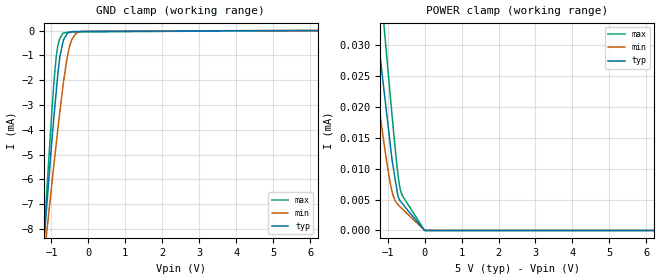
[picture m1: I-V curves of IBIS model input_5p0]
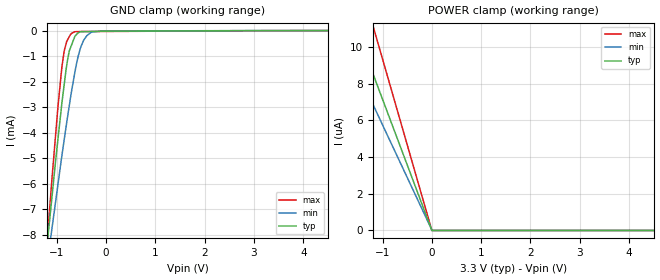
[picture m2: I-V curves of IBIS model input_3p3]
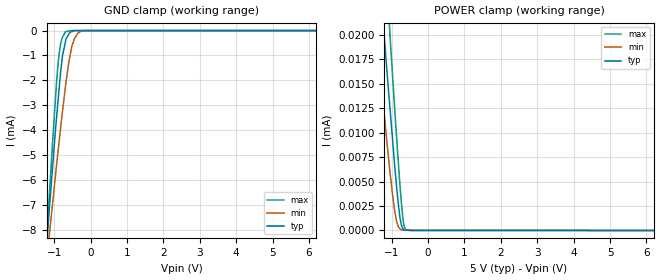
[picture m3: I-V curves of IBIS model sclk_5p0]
|Texas Instruments Incorporated
| 3 Phase Motor Driver-IC for Automotive Safety Applications
| Marketing part#   Digital Voltage Range   Package-type   #pins
| DRV3201QPAPQ1   1.72V-5.5V   HTQFP   64
[IBIS Ver]   4.1
[File name]   drv3201.ibs
[File Rev]   1.0
[Date]   2/26/2013
[Source]
| Texas Instruments Incorporated.
| Analog-eLab Design Center, HPA
| 12500 TI Blvd
| Dallas, TX -75243
[Notes]   Revision History:
| Rev 1.0: 2/26/2013
| - Initial version of the model
| - Model generated from simulations in TISPICE
| - Model matched to SPICE simulation
| - C_comp although listed in numerical order of value are
|   obtained from varying PVT conditions. For PVT conditions for
|   each specific value refer the buffer description under
|   respective [Model]. IBIS model user is responsible for using
|   appropriate C_comp to simulate for Signal Integrity.
| - Model names with a trailing _3p3 contains the model for 3.3V
|   [3.0V and 3.6V]. Model names with a trailing _5 contains the
|   model for 5.0V [4.5V and 5.5V].
[Disclaimer]
| This model is designed as an aid for customers of Texas Instruments.
| TI and its licensors and suppliers make no warranties, either expressed
| or implied, with respect to this  model, including the warranties of
| merchantability or fitness for a particular purpose. The model is
| provided solely on an "as is" basis. The entire risk as to its quality
| and performance is with the customer.
|*  EXCEPTION:   *
|*  - For model en_*, there will be a leakage current in the power clamp   *
|*   I-V Table because of the pull down resistor RES_P1H (200K) and the   *
|*   diode DIO_Z_CB_MV1 connected to pad.   *
|*  - For model input_*, there will be a leakage current in the ground   *
|*   clamp I-V Table because of the  pull-up resistor RES_P1H (140K)   *
|*   connected to pad.   *
|*  - For model sclk_*, there will be a leakage current in the power clamp  *
|*   I-V Table because of the esd transistor NPN_ESD_5A connected to pad.  *
|*  - For model sdi_*, there will be a leakage current in the power clamp   *
|*   I-V Table because of the esd transistor NPN_ESD_5A connected to pad.  *
[Copyright]
(C) Copyright 2013 Texas Instruments Incorporated.All rights reserved.
|   DRV3201
[Component]   DRV3201
[Manufacturer]   TI
[Package]   |64 HTQFP   -  PAP package
|   typ   min   max
R_pkg   0.07164   0.06786   0.07759
L_pkg   3.33226nH   3.17288nH   3.57776nH
C_pkg   0.48700pF   0.46154pF   0.50805pF
[Pin]  signal_name   model_name   R_pin   L_pin   C_pin
1   VSH   NC   0.07673   3.54889nH  0.46840pF
2   SLS3   POWER   0.07311   3.39626nH  0.51137pF
3   GLS3   POWER   0.07001   3.27956nH  0.49926pF
4   SHS3   POWER   0.06923   3.24062nH  0.49391pF
5   GHS3   POWER   0.06747   3.17175nH  0.48377pF
6   PGND   GND   0.06709   3.14589nH  0.47600pF
7   SLS2   POWER   0.06644   3.11361nH  0.47461pF
8   GLS2   POWER   0.06615   3.10081nH  0.46390pF
9   SHS2   POWER   0.06619   3.10253nH  0.46433pF
10   GHS2   POWER   0.06676   3.12576nH  0.48040pF
11   GNDA   GND   0.06824   3.18796nH  0.48872pF
12   SCTH   NC   0.07010   3.26538nH  0.49431pF
13   SLS1   POWER   0.07197   3.33861nH  0.50666pF
14   GLS1   POWER   0.07533   3.46841nH  0.51599pF
15   SHS1   POWER   0.07680   3.52858nH  0.52091pF
16   GHS1   POWER   0.08171   3.72851nH  0.48358pF
17   PH1C   PH   0.07690   3.56798nH  0.46154pF
18   PH2C   PH   0.07539   3.49007nH  0.50339pF
19   PH3C   PH   0.07491   3.46547nH  0.50805pF
20   GNDA   GND   0.07195   3.34941nH  0.50551pF
21   DRVOFF   INPUT   0.06967   3.26125nH  0.48761pF
22   SCLK   SCLK   0.06998   3.25832nH  0.48236pF
23   GNDL   GND   0.06864   3.20087nH  0.48096pF
24   NCS   INPUT   0.06798   3.17337nH  0.46659pF
25   SDI   SDI   0.06796   3.17288nH  0.46520pF
26   SDO   SDO   0.06786   3.17339nH  0.47390pF
27   GNDA   GND   0.06804   3.19040nH  0.48153pF
28   VS   POWER   0.06907   3.23961nH  0.48931pF
29   BOOST   POWER   0.06978   3.27269nH  0.49651pF
30   SW   POWER   0.03802   3.09902nH  0.55354pF
31   GNDLS_B   GND   0.03874   3.15006nH  0.56153pF
32   NC   NC   0.07644   3.55028nH  0.47304pF
33   NC   NC   0.07611   3.53711nH  0.46336pF
34   B_EN   INPUT   0.07412   3.44194nH  0.50787pF
35   CSM   SDI   0.07078   3.31667nH  0.49695pF
36   EN   EN   0.07096   3.31071nH  0.49365pF
37   RSTN   INPUT   0.06872   3.22236nH  0.48158pF
38   ERR   ERR   0.07110   3.29339nH  0.48566pF
39   GNDA   GND   0.06849   3.19000nH  0.48290pF
40   VCC5   NC   0.06688   3.12853nH  0.46693pF
41   TEST(GND)   NC   0.06665   3.11990nH  0.46778pF
42   VCC3   NC   0.03537   2.85634nH  0.51702pF
43   AMUX(GND)   GND   0.06623   3.11968nH  0.47403pF
44   ADREF   NC   0.06627   3.13372nH  0.48099pF
45   GNDL   GND   0.06693   3.16429nH  0.48921pF
46   O4   NC   0.06838   3.22606nH  0.49485pF
47   O3   NC   0.07039   3.30331nH  0.50075pF
48   O2   NC   0.07861   3.61686nH  0.47279pF
49   IN2   NC   0.08054   3.68122nH  0.47742pF
50   IP2   NC   0.07690   3.52768nH  0.52252pF
51   GNDA   GND   0.07282   3.37580nH  0.51523pF
52   RO   NC   0.06992   3.26214nH  0.50012pF
53   RI   NC   0.06865   3.20956nH  0.48695pF
54   IP1   NC   0.06779   3.16608nH  0.47853pF
55   O1   NC   0.06756   3.14757nH  0.47304pF
56   IN1   NC   0.06757   3.14359nH  0.46926pF
57   GNDA   GND   0.06819   3.16549nH  0.47185pF
58   VDDIO   POWER   0.06871   3.18793nH  0.47574pF
59   IHS3   SDI   0.06892   3.20623nH  0.47992pF
60   ILS3   SDI   0.07066   3.28064nH  0.48755pF
61   IHS2   SDI   0.07071   3.29082nH  0.49336pF
62   ILS2   SDI   0.07325   3.39194nH  0.50262pF
63   IHS1   SDI   0.07376   3.41784nH  0.50532pF
64   ILS1   SDI   0.07759   3.57776nH  0.46991pF
|   Model Selectors
[Model Selector] INPUT
input_3p3  3.3V digital input
input_5p0  5.0V digital input
[Model Selector] SCLK
sclk_3p3  3.3V digital input
sclk_5p0  5.0V digital input
[Model Selector] SDI
sdi_3p3  3.3V digital input
sdi_5p0  5.0V digital input
[Model Selector] EN
en_3p3  3.3V digital input
en_5p0  5.0V digital input
[Model Selector] PH
ph_3p3  3.3V digital output
ph_5p0  5.0V digital output
[Model Selector] ERR
err_3p3  3.3V digital output
err_5p0  5.0V digital output
[Model Selector] SDO
sdo_3p3  3.3V digital output
sdo_5p0  5.0V digital output
| Models and submodels in the file (14): input_5p0 (Input), input_3p3 (Input), sclk_5p0 (Input), sclk_3p3 (Input), en_5p0 (Input), en_3p3 (Input), sdi_5p0 (Input), sdi_3p3 (Input), ph_5p0 (Output), ph_3p3 (Output), err_5p0 (Output), err_3p3 (Output), sdo_5p0 (Output), sdo_3p3 (Output)
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|   input_5p0 Model
[Model]   input_5p0
Model_type   Input
Vinl = 1.5
Vinh = 3.5
|   typ   min   max
|   (nom PVT)   (fast PVT)   (slow PVT)
C_comp   4.496e-13   4.401e-13   4.837e-13
| Where nom  PVT is Nominal Process, 5V, 27C
|   Fast PVT is Strong Process,  5.5V, -40C
|   Slow PVT is Weak Process,   4.5V, 150C
[Voltage Range]   5   4.5   5.5
[Temperature Range]   27   150   -40
[Power Clamp Reference]   5   4.5   5.5
[GND Clamp Reference]   0   0   0
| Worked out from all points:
|   GND clamp passes 1 mA (typ) near -0.76 V on its own axis
[GND Clamp]
|   Voltage   I(typ)   I(min)   I(max)
-5V       -87.91mA   -68.74mA   -109.8mA
-1.21V    -8.701mA   -9.359mA   -8.617mA
-1.139V   -7.31mA    -8.314mA   -6.835mA
-1.083V   -6.272mA   -7.533mA   -5.494mA
-940.5mV  -3.622mA   -5.516mA   -2.263mA
-869mV    -2.453mA   -4.558mA   -1.045mA
-770mV    -1.039mA   -3.255mA   -318.7uA
-687.5mV  -468.2uA   -2.242mA   -104.3uA
-513mV    -80.01uA   -652.5uA   -56.2uA
-346.5mV  -38.89uA   -131.6uA   -54.55uA
-202.5mV  -37.57uA   -32.73uA   -53.21uA
10V       0A         0A         0A
[POWER Clamp]
|   Voltage   I(typ)   I(min)   I(max)
-5V       244.6uA    202.3uA    308.1uA
-1.566V   48.38uA    35.32uA    65.5uA
-1.373V   37.57uA    26.3uA     51.98uA
-1.175V   26.68uA    17.38uA    38.37uA
-1.098V   22.63uA    14.09uA    33.11uA
-1.078V   21.59uA    13.27uA    31.73uA
-891mV    11.91uA    6.548uA    19.26uA
-720mV    5.513uA    4.176uA    9.035uA
-671mV    4.865uA    3.873uA    6.977uA
-594mV    4.287uA    3.425uA    5.569uA
-84.44fV  0A         25.24nA    0A
10V       0A         0A         0A
|   input_3p3 Model
[Model]   input_3p3
Model_type   Input
Vinl = 0.99
Vinh = 2.31
|   typ   min   max
|   (nom PVT)   (fast PVT)   (slow PVT)
C_comp   4.837e-13   4.556e-13   5.145e-13
| Where nom  PVT is Nominal Process, 3.3V, 27C
|   Fast PVT is Strong Process,  3.6V, -40C
|   Slow PVT is Weak Process,   3V, 150C
[Voltage Range]   3.3   3   3.6
|Junction Temperature
[Temperature Range]   27   150   -40
[Power Clamp Reference]   3.3   3   3.6
[GND Clamp Reference]   0   0   0
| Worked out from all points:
|   GND clamp passes 1 mA (typ) near -0.77 V on its own axis
[GND Clamp]
|   Voltage   I(typ)   I(min)   I(max)
-3.3V     -51.91mA   -41.45mA   -64.06mA
-1.181V   -8.13mA    -8.949mA   -7.907mA
-1.094V   -6.469mA   -7.714mA   -5.739mA
-975.6mV  -4.253mA   -6.028mA   -2.981mA
-896.4mV  -2.845mA   -4.904mA   -1.432mA
-849.6mV  -2.122mA   -4.283mA   -802.6uA
-745.8mV  -794.5uA   -2.94mA    -239uA
-633.6mV  -230.5uA   -1.641mA   -44.95uA
-561mV    -84.79uA   -969.8uA   -40.68uA
-456mV    -41.05uA   -382.5uA   -37.85uA
-285mV    -34.46uA   -56.96uA   -36.25uA
6.6V      0A         0A         0A
[POWER Clamp]
|   Voltage   I(typ)   I(min)   I(max)
-3.3V     62.42uA    54.6uA     71.62uA
-2.19V    15.65uA    12.57uA    20.44uA
-897.6mV  6.409uA    5.161uA    8.375uA
-33.83fV  0A         25.22nA    0A
6.6V      0A         0A         0A
|   sclk_5p0 Model
[Model]   sclk_5p0
Model_type   Input
Vinl = 1.5
Vinh = 3.5
|   typ   min   max
|   (nom PVT)   (fast PVT)   (slow PVT)
C_comp   4.496e-13   4.401e-13   4.837e-13
| Where nom  PVT is Nominal Process, 5V, 27C
|   Fast PVT is Strong Process,  5.5V, -40C
|   Slow PVT is Weak Process,   4.5V, 150C
[Voltage Range]   5   4.5   5.5
|Junction Temperature
[Temperature Range]   27   150   -40
[Power Clamp Reference]   5   4.5   5.5
[GND Clamp Reference]   0   0   0
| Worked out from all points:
|   GND clamp passes 1 mA (typ) near -0.77 V on its own axis
[GND Clamp]
|   Voltage   I(typ)   I(min)   I(max)
-5V       -87.84mA   -68.69mA   -109.7mA
-1.21V    -8.657mA   -9.326mA   -8.555mA
-1.139V   -7.267mA   -8.282mA   -6.774mA
-1.083V   -6.228mA   -7.501mA   -5.433mA
-940.5mV  -3.58mA    -5.486mA   -2.203mA
-869mV    -2.411mA   -4.528mA   -985.8uA
-770mV    -998.3uA   -3.225mA   -260.2uA
-687.5mV  -427.6uA   -2.212mA   -46.56uA
-513mV    -40.64uA   -623.8uA   -122.7nA
-346.5mV  -716.2nA   -103.9uA   0A
-202.5mV  -418.6nA   -5.828uA   0A
10V       0A         0A         0A
[POWER Clamp]
|   Voltage   I(typ)   I(min)   I(max)
-5V       211.5uA    175.9uA    264.8uA
-1.809V   49.78uA    36.93uA    66.43uA
-1.375V   28.23uA    18.77uA    39.82uA
-1.238V   21.58uA    13.24uA    31.49uA
-1.14V    16.86uA    9.466uA    25.68uA
-1.044V   12.47uA    5.95uA     19.95uA
-900mV    5.936uA    1.652uA    11.58uA
-830mV    3.175uA    547.7nA    7.738uA
-742.5mV  746.6nA    82.4nA     3.289uA
-660mV    46.92nA    33.23nA    496.6nA
-500.5mV  13.7nA     30.45nA    0A
10V       0A         0A         0A
